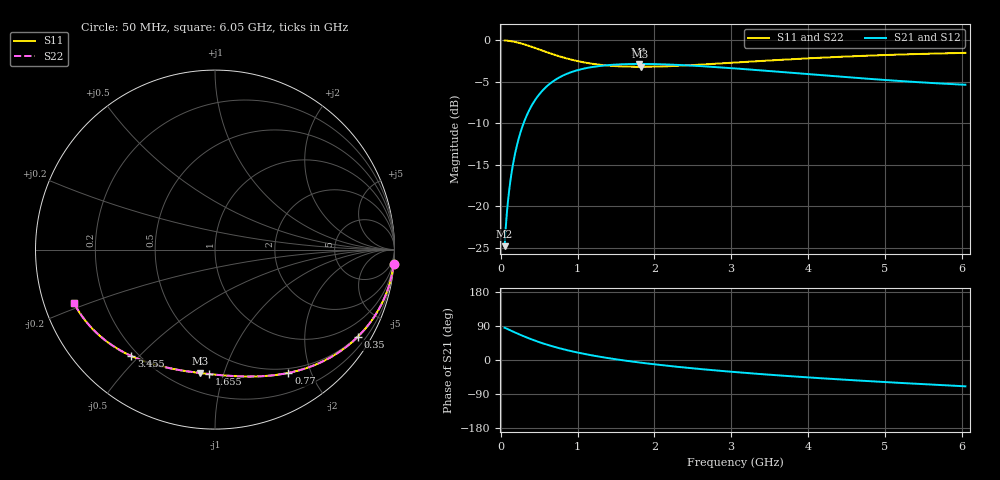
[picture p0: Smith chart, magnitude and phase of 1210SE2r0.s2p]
! AVX Thin Film Operation		Date: August 2001
! Description: Accu-P® Series, Thin Film, SMD, RF Capacitor
! Part Number: 12101J2R0ABT
! 50 MHz  -  6.05 GHz
! Serial Measurements
# mhz S db R 50
!	S11		S21		S12		S22
!	dB	Phase	dB	Phase	dB	Phase	dB	Phase
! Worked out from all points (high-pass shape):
!   401 points, 50 MHz to 6.05 GHz, reference 50 ohm
!   highest |S21| = -2.84 dB at 1.805 GHz (marker M1); lowest = -24.8 dB at 50 MHz (marker M2)
!   |S21| within 3 dB of the highest: 564.6 MHz to end of sweep
!   lowest |S11| = -3.2 dB at 1.82 GHz (marker M3), VSWR 5.51, Z = 15.8 - j41.8 ohm
!   |S11| at or under -10 dB: nowhere
!   |S22| runs from -3.2 to 0.0 dB; largest |S21 - S12| = 0
!   S11 on the Smith chart (normalised r, x): 50 MHz: 0, -24; 350 MHz: 0.47, -3.49; 770 MHz: 0.44, -1.67; 1.655 GHz: 0.34, -0.90; 3.455 GHz: 0.17, -0.47; 6.05 GHz: 0.09, -0.18
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50  -0.01 -4.8  -24.79 85.2  -24.79 85.2  -0.01 -4.8
65  -0.02 -6.2  -22.53 83.8  -22.53 83.8  -0.02 -6.2
110  -0.07 -10.4  -18.02 79.6  -18.02 79.6  -0.07 -10.4
140  -0.11 -13.2  -15.99 76.8  -15.99 76.8  -0.11 -13.2
170  -0.16 -16.0  -14.38 74.0  -14.38 74.0  -0.16 -16.0
245  -0.32 -22.7  -11.45 67.3  -11.45 67.3  -0.32 -22.7
350  -0.61 -31.5  -8.80 58.5  -8.80 58.5  -0.61 -31.5
440  -0.90 -38.5  -7.29 51.5  -7.29 51.5  -0.90 -38.5
545  -1.25 -45.8  -6.03 44.1  -6.03 44.1  -1.25 -45.9
770  -1.95 -59.3  -4.43 30.7  -4.43 30.7  -1.95 -59.3
1055  -2.60 -72.6  -3.46 17.4  -3.46 17.4  -2.60 -72.6
1325  -2.98 -82.6  -3.05 7.4  -3.05 7.4  -2.98 -82.6
1655  -3.17 -92.6  -2.86 -2.6  -2.86 -2.6  -3.17 -92.6
1805  -3.19 -96.5  -2.84 -6.6  -2.84 -6.6  -3.19 -96.6
1820  -3.19 -96.9  -2.84 -6.9  -2.84 -6.9  -3.19 -96.9
2060  -3.15 -102.7  -2.88 -12.7  -2.88 -12.7  -3.15 -102.7
2540  -2.96 -112.7  -3.07 -22.7  -3.07 -22.7  -2.96 -112.7
3050  -2.68 -121.8  -3.38 -31.8  -3.38 -31.8  -2.68 -121.8
3455  -2.45 -128.2  -3.67 -38.2  -3.67 -38.2  -2.45 -128.2
4055  -2.14 -136.6  -4.11 -46.6  -4.11 -46.6  -2.14 -136.6
5060  -1.75 -148.8  -4.81 -58.9  -4.81 -58.9  -1.75 -148.8
6050  -1.51 -159.4  -5.35 -69.5  -5.35 -69.5  -1.51 -159.4
